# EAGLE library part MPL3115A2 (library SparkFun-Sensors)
NXP MPL3115A2 Digital Altimeter/Pressure Sensor The MPL3115A2 is a compact piezoresistive absolute pressure sensor with an I2C interface. MPL3115 has a wide operating range of 20kPa to 110 kPa, a range that covers all surface elevations on Earth. The fully internally compensated MEMS in conjunction with an embedded high resolution 24-bit equivalent ADC provide accurate pressure [Pascals] /altitude [meters] and temperature [degrees Celsius] data. Datasheet SparkFun Products SparkFun Altitude/Pressure Sensor Breakout - MPL3115A2 (SEN-11084) SparkFun Weather Shield (DEV-12081) SparkFun Photon Weather Shield (DEV-13630)
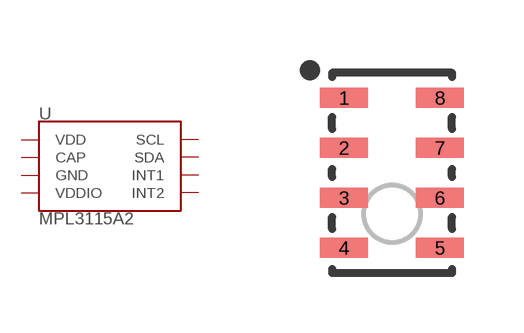
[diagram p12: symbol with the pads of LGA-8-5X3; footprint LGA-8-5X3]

Designator prefix U

## MPL3115A2 (PROD_ID: IC-10869)  [LGA-8-5X3]
1  VDD  pwr
2  CAP  pwr
3  GND  pwr
4  VDDIO  pwr
5  INT2  out
6  INT1  out
7  SDA
8  SCL

## Footprint LGA-8-5X3 (pad centres in mm)
8-Pin Land Grid Array (LGA) (5 x 3 mm) Datasheet Specifications: Pin Count: 8 Area: 5.0 x 3.0 x 1.2 mm Pitch: 1.25 mm Devices Using: MPL115A MPL3115A2
smd 1.2 x 0.5: 1 -1.2,1.875; 2 -1.2,0.625; 3 -1.2,-0.625; 4 -1.2,-1.875; 5 1.2,-1.875; 6 1.2,-0.625; 7 1.2,0.625; 8 1.2,1.875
